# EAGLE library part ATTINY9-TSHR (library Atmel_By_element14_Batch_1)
Microcontroller
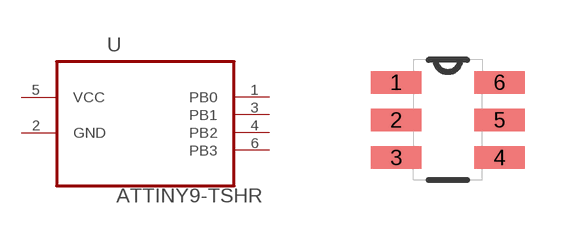
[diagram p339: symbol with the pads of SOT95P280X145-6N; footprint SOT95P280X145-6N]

Designator prefix U

## ATTINY9-TSHR (DESCRIPTION: Microcontroller; MPN: ATTINY9-TSHR; OC_FARNELL: 1841629; OC_NEWARK: 12T1345; PACKAGE: SOT563-6; SUPPLIER: ATMEL)  [SOT95P280X145-6N]
1  PB0
2  GND  pas
3  PB1
4  PB2
5  VCC  pwr
6  PB3

## Footprint SOT95P280X145-6N (pad centres in mm)
smd 1.27 x 0.559: 1 -1.295,0.94; 2 -1.295,0; 3 -1.295,-0.94; 4 1.295,-0.94; 5 1.295,0; 6 1.295,0.94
